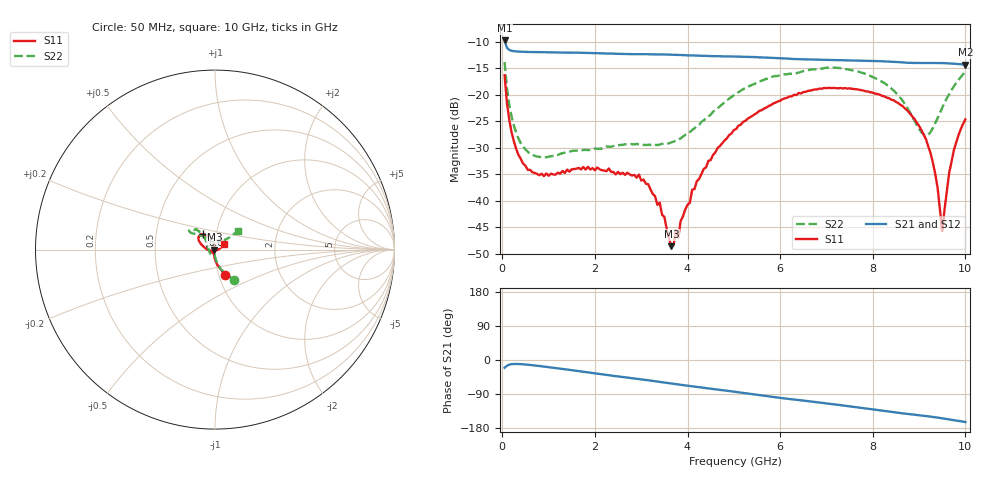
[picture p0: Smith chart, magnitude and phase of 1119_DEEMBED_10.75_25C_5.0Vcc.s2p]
!Hittite Microwave Corp.
!Digital Attenuator/PhaseShifter Rev 1.4.0
!Filename: C:\DATA\DATA\1119_DEEMBED_10.75_25C_5.0Vcc.s2p
!VNA ID: Agilent Technologies,N5224A,MY51441122,A.10.45.03
!Device type:
!2 Port Calibration.
!Temp(C): 25
!Lot Number:
!Serial Number:
!Operator:
!Misc:
!Attenuator:  10.750
# GHZ S DB R 50.0
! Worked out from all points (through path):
!   200 points, 50 MHz to 10 GHz, reference 50 ohm
!   highest |S21| = -9.77 dB at 50 MHz (marker M1); lowest = -14.3 dB at 10 GHz (marker M2)
!   group delay of S21, straight-line fit = 43.7 ps
!   lowest |S11| = -48.5 dB at 3.65 GHz (marker M3), VSWR 1.01, Z = 49.6 - j0.0301 ohm
!   |S11| at or under -10 dB: start of sweep to end of sweep
!   |S22| runs from -31.8 to -13.9 dB; largest |S21 - S12| = 0.00082
!   S11 on the Smith chart (normalised r, x): 50 MHz: 1.07, -0.31; 6.6 GHz: 0.86, +0.15; 10 GHz: 1.10, +0.07
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0.05  -16.31 -68.0  -9.77 -20.4  -9.77 -20.4  -13.87 -58.0
0.1  -21.51 -81.7  -11.15 -15.2  -11.15 -15.2  -18.66 -73.0
0.2  -27.05 -93.6  -11.71 -11.0  -11.71 -11.1  -24.09 -83.8
0.55  -34.16 -113.9  -11.93 -12.4  -11.93 -12.5  -30.74 -94.5
1.75  -33.61 -129.6  -12.10 -31.0  -12.11 -31.0  -30.40 -111.4
2.95  -35.05 -118.7  -12.35 -50.3  -12.36 -50.3  -29.34 -148.6
3.4  -40.33 -133.9  -12.40 -57.7  -12.41 -57.8  -29.36 -169.7
3.65  -48.53 -175.4  -12.47 -61.9  -12.48 -62.0  -28.99 177.2
3.75  -45.52 145.1  -12.48 -63.7  -12.49 -63.7  -28.62 171.7
3.8  -46.93 132.4  -12.50 -64.5  -12.50 -64.6  -28.44 168.0
3.85  -43.83 125.2  -12.52 -65.3  -12.52 -65.4  -28.23 165.4
4.2  -36.31 99.0  -12.64 -71.0  -12.65 -71.1  -25.92 147.5
5.05  -26.46 104.9  -12.81 -84.3  -12.83 -84.4  -19.80 129.3
6.6  -19.28 128.9  -13.34 -108.5  -13.35 -108.6  -15.37 139.7
6.7  -19.11 130.5  -13.35 -110.1  -13.36 -110.1  -15.23 140.2
8.35  -20.64 154.9  -13.75 -136.0  -13.75 -136.0  -18.43 137.0
9.15  -28.41 -176.9  -14.00 -147.8  -14.02 -147.8  -27.67 88.0
9.35  -34.96 -156.9  -14.00 -151.2  -14.02 -151.2  -25.34 57.9
9.5  -45.66 -83.7  -14.03 -153.9  -14.04 -154.0  -22.40 45.3
9.65  -34.70 1.5  -14.09 -156.8  -14.11 -156.8  -19.88 40.4
9.75  -30.45 15.4  -14.15 -158.8  -14.16 -158.8  -18.42 39.3
10  -24.64 32.4  -14.33 -163.6  -14.34 -163.6  -15.69 39.9
